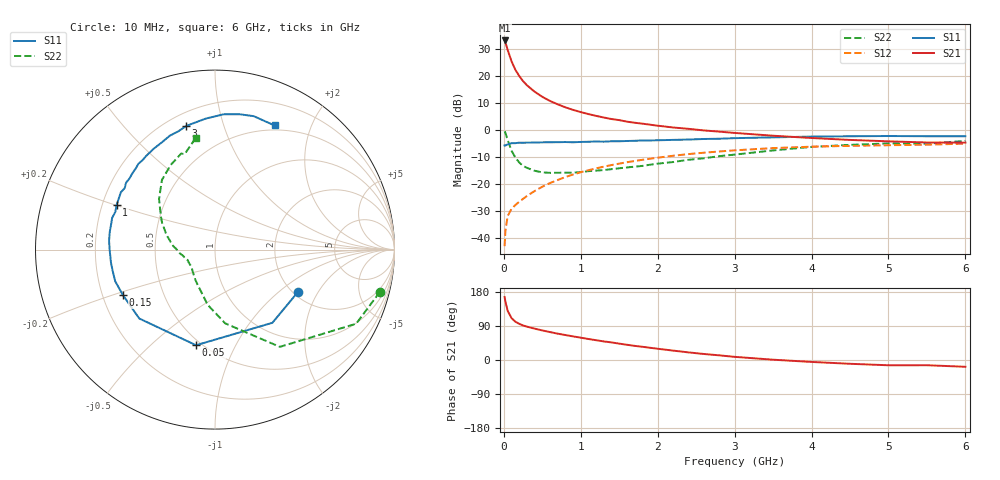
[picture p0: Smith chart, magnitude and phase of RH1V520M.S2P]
! SIEMENS Small Signal Semiconductors
! BFR106
! Si NPN RF Bipolar Junction Transistor in SOT23
! VCE = 1.5 V  IC = 20 mA
! Common Emitter S-Parameters:  August  1996
# GHz  S  MA  R  50
!  f  S11  S21  S12  S22
! GHz  MAG  ANG  MAG  ANG  MAG  ANG  MAG  ANG
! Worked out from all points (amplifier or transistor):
!   36 points, 10 MHz to 6 GHz, reference 50 ohm
!   highest |S21| = 33.0 dB at 10 MHz (marker M1)
!   |S21| within 3 dB of that: start of sweep to 44.74 MHz
!   unconditionally stable (mu >= 1): 345.3 MHz to 2.771 GHz; 4.643 GHz to end of sweep
!   at 250 MHz: K = 0.91, MSG = 21.7 dB, |S12| = -25.4 dB
!   at 1.4 GHz: K = 1.08, MAG = 6.7 dB, |S12| = -12.9 dB
!   at 6 GHz: K = 1.02, MAG = -0.7 dB, |S12| = -5.0 dB
!   S11 on the Smith chart (normalised r, x): 10 MHz: 2.10, -1.37; 50 MHz: 0.47, -0.71; 150 MHz: 0.29, -0.22; 1 GHz: 0.26, +0.20; 3 GHz: 0.27, +0.76; 6 GHz: 0.44, +1.50
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0.01  0.5183 -27.4  44.82 166.1  0.0072 81.3  0.9484 -14.4
0.02  0.5182 -51.9  41.6 154.6  0.0137 71.8  0.8882 -27.7
0.05  0.5431 -101.2  29.96 129.5  0.0259 54.4  0.6514 -56.3
0.1  0.5705 -137.7  18.48 110.5  0.0352 49.3  0.415 -82.1
0.15  0.572 -153.6  12.89 101.0  0.0414 49.8  0.3103 -97.6
0.2  0.5832 -162.3  9.917 95.4  0.0475 53.4  0.2519 -107.1
0.25  0.5825 -168.5  7.967 91.1  0.0537 55.5  0.2177 -116.6
0.3  0.5841 -172.8  6.69 88.0  0.0606 58.1  0.2006 -123.1
0.4  0.5869 -179.8  5.085 82.8  0.0749 60.9  0.1772 -133.7
0.5  0.5923 175.2  4.088 78.0  0.0899 62.4  0.1652 -141.4
0.6  0.5945 170.5  3.436 73.7  0.105 63.3  0.1621 -146.5
0.7  0.5957 166.3  2.976 69.5  0.1198 63.2  0.1627 -151.1
0.8  0.5997 162.9  2.62 65.9  0.1355 62.7  0.1632 -155.7
1  0.6022 155.6  2.139 58.9  0.1664 61.4  0.1678 -161.2
1.1  0.6069 152.1  1.965 55.4  0.1812 60.4  0.1742 -164.0
1.6  0.6269 137.2  1.426 40.2  0.2544 53.8  0.204 -176.7
2.2  0.657 121.7  1.113 24.8  0.3346 44.6  0.2564 168.7
3  0.7072 103.1  0.883 8.3  0.4216 31.5  0.3514 148.9
3.5  0.7317 94.1  0.784 0.8  0.4636 23.7  0.4203 137.9
4.5  0.7664 79.7  0.656 -10.0  0.5097 9.0  0.5319 117.7
5.5  0.7673 68.2  0.588 -13.8  0.5355 0.1  0.5583 107.6
6  0.7675 64.4  0.585 -17.9  0.5599 -6.8  0.6299 99.9
